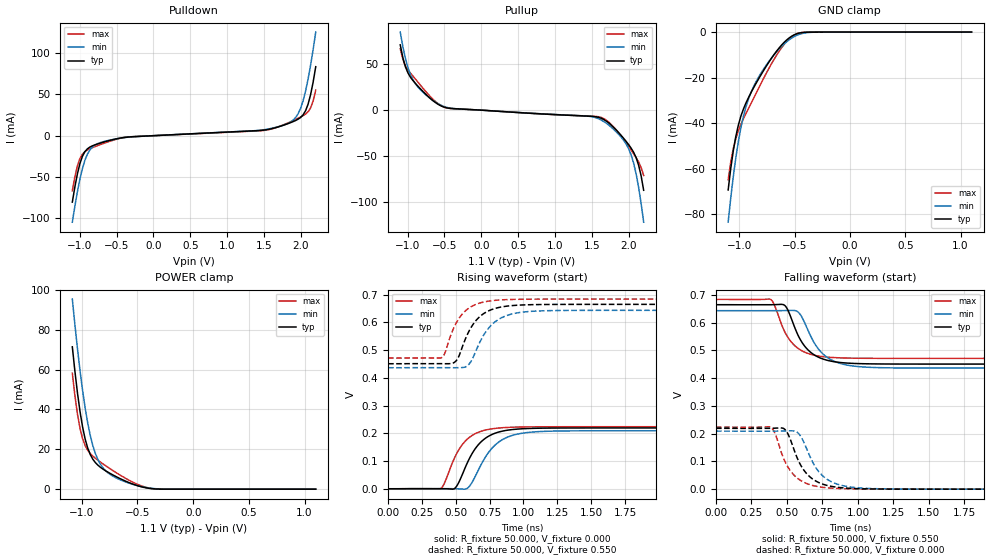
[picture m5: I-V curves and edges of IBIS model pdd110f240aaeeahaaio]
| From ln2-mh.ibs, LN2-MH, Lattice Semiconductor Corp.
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|   Model pdd110f240aaeeahaaio
[Model] pdd110f240aaeeahaaio
| Clamp models do not include dynamic input termination. Please refer to
| the pdd110axxxaaeeahaain model for input termination.
Model_type I/O
Polarity   Non-Inverting
Enable   Active-Low
Vinl =  0.700V
Vinh =  0.900V
Vmeas =  0.550V
Cref =  20.000pF
Rref =  50.000
Vref =  0.600V
C_comp   2.000pF   1.500pF   2.500pF
[Temperature Range]   25.000   0.125k   -40.000
[Voltage Range]   1.100V   1.070V   1.130V
[C Comp Corner]
C_comp   2.000pF   1.500pF   2.500pF
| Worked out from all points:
|   slope of the pulldown table from 0 to 0.165 V, typ, clamps not added: 226 ohm
|   slope of the pullup table from 0 to 0.165 V, typ, clamps not added: 189 ohm
|   GND clamp passes 1 mA (typ) near -0.49 V on its own axis
|   POWER clamp passes 1 mA (typ) near -0.45 V on its own axis
|   rising waveform, R_fixture 50.000, V_fixture 0.000: 20-80 % time 160ps typ, 174ps min, 149ps max; typ from 0 V to 0.219 V
|   rising waveform, R_fixture 50.000, V_fixture 0.550: 20-80 % time 145ps typ, 159ps min, 135ps max; typ from 0.451 V to 0.665 V
|   falling waveform, R_fixture 50.000, V_fixture 0.550: 20-80 % time 141ps typ, 153ps min, 134ps max; typ from 0.665 V to 0.451 V
|   falling waveform, R_fixture 50.000, V_fixture 0.000: 20-80 % time 136ps typ, 146ps min, 130ps max; typ from 0.219 V to 0 V
[Pulldown]
|Voltage   I(typ)   I(min)   I(max)
-1.1V     -80.41mA   -104.7mA   -66.6mA
-1.032V   -46.71mA   -68.33mA   -36.85mA
-930mV    -19.42mA   -29.84mA   -19.32mA
-862mV    -13.81mA   -17.24mA   -15.74mA
-760mV    -10.08mA   -9.781mA   -12.09mA
-352mV    -1.714mA   -1.878mA   -1.639mA
1.518V    7.039mA    7.489mA    6.6mA
1.892V    16.99mA    18.71mA    18.2mA
1.96V     19.93mA    26.39mA    21.06mA
2.028V    25.15mA    42.13mA    24.19mA
2.13V     49.57mA    85.28mA    33.6mA
2.2V      83.5mA     125.4mA    55.21mA
[Pullup]
|Voltage   I(typ)   I(min)   I(max)
-1.1V     71.14mA    85.08mA    66.87mA
-1.03V    47.19mA    56.36mA    48.33mA
-928mV    32.35mA    33.12mA    37.14mA
-792mV    20.37mA    19.56mA    23.9mA
-554mV    4.909mA    5.643mA    5.273mA
1.452V    -6.529mA   -6.64mA    -6.444mA
1.724V    -13.8mA    -16.09mA   -12.89mA
1.928V    -30.66mA   -32.78mA   -31.94mA
2.03V     -41.41mA   -48.75mA   -43.49mA
2.098V    -51.87mA   -69.53mA   -51.8mA
2.132V    -60.12mA   -84.3mA    -56.57mA
2.2V      -87.31mA   -122.1mA   -71.2mA
[GND_clamp]
|Voltage   I(typ)   I(min)   I(max)
-1.1V     -69.42mA   -83.58mA   -64.91mA
-1.054V   -52.28mA   -63.71mA   -51.34mA
-1.008V   -40.93mA   -48.17mA   -43.43mA
-962mV    -33.84mA   -37.03mA   -38.1mA
-916mV    -28.78mA   -29.39mA   -33.57mA
-847mV    -22.46mA   -21.74mA   -26.86mA
-778mV    -16.75mA   -16.15mA   -20.21mA
-663mV    -8.418mA   -8.698mA   -10.2mA
-571mV    -3.463mA   -4.234mA   -4.089mA
-502mV    -1.179mA   -1.94mA    -1.255mA
-410mV    -105.5uA   -402.4uA   -63.37uA
1.1V      0A         0A         0A
[POWER_clamp]
|Voltage   I(typ)   I(min)   I(max)
-1.085V   71.41mA    95.35mA    58.18mA
-1.062V   59.23mA    82.55mA    46.99mA
-1.039V   48.36mA    70.56mA    37.71mA
-1.016V   38.97mA    59.53mA    30.53mA
-970mV    25.17mA    40.76mA    21.88mA
-924mV    17.37mA    26.93mA    17.87mA
-901mV    15.03mA    21.86mA    16.59mA
-855mV    12.01mA    14.79mA    14.5mA
-763mV    8.448mA    8.108mA    10.89mA
-533mV    2.369mA    2.267mA    3.272mA
-349mV    143.9uA    291.4uA    171.3uA
1.1V      0A         0A         0A
[Ramp]
| variable   typ   min   max
dV/dt_r   0.132/0.160n   0.125/0.174n   0.134/0.149n
dV/dt_f   0.119/0.150n   0.117/0.169n   0.115/0.140n
R_load = 50.000
[Rising Waveform]
R_fixture = 50.000
V_fixture = 0.000
V_fixture_min = 0.000
V_fixture_max = 0.000
|  time   V(typ)   V(min)   V(max)
0s        2.527uV    12.65uV    1.11uV
389ps     346.7uV    169.2uV    728.8uV
495ps     2.515mV    -39.9uV    115.4mV
578ps     85.34mV    -195.5uV   175.5mV
618ps     124.6mV    20.99mV    191.2mV
698ps     174mV      96.7mV     208.8mV
779ps     198mV      152mV      216.8mV
880ps     210.9mV    185.5mV    221mV
1.36ns    219.1mV    208.6mV    223.5mV
10ns      219.3mV    209.1mV    223.6mV
[Rising Waveform]
R_fixture = 50.000
V_fixture = 0.550
V_fixture_min = 0.534
V_fixture_max = 0.568
|  time   V(typ)   V(min)   V(max)
0s        450.6mV    436.2mV    471.2mV
398ps     450.8mV    436.4mV    473.3mV
503ps     461.4mV    436.2mV    597.2mV
574ps     543.1mV    439.7mV    642.3mV
617ps     584.4mV    462.6mV    657.1mV
691ps     625.9mV    540.7mV    671.2mV
769ps     646.5mV    592.6mV    678mV
871ps     657.8mV    623.3mV    681.6mV
1.331ns   664.5mV    642.8mV    683.7mV
10ns      664.7mV    643.2mV    683.7mV
[Falling Waveform]
R_fixture = 50.000
V_fixture = 0.550
V_fixture_min = 0.534
V_fixture_max = 0.568
|  time   V(typ)   V(min)   V(max)
0s        664.7mV    643.2mV    683.7mV
385ps     664.6mV    643.1mV    683.6mV
411ps     664.8mV    643.2mV    663.6mV
486ps     661.2mV    643.6mV    565.5mV
568ps     565.8mV    641.6mV    511.3mV
637ps     507.8mV    585.4mV    491.1mV
723ps     475.2mV    504.1mV    479.6mV
857ps     457.5mV    456mV      473.5mV
1.331ns   450.8mV    436.6mV    471.2mV
10ns      450.6mV    436.2mV    471.2mV
[Falling Waveform]
R_fixture = 50.000
V_fixture = 0.000
V_fixture_min = 0.000
V_fixture_max = 0.000
|  time   V(typ)   V(min)   V(max)
0s        219.3mV    209.1mV    223.6mV
386ps     219.4mV    209.1mV    223mV
417ps     219.9mV    209.1mV    199.5mV
488ps     213.8mV    210mV      97.41mV
564ps     122.8mV    207.5mV    43.7mV
627ps     63.04mV    159.7mV    22.96mV
722ps     24.34mV    64.36mV    8.925mV
863ps     6.321mV    16.69mV    2.313mV
1.313ns   169.4uV    422.4uV    71.99uV
10ns      2.527uV    12.65uV    1.11uV
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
